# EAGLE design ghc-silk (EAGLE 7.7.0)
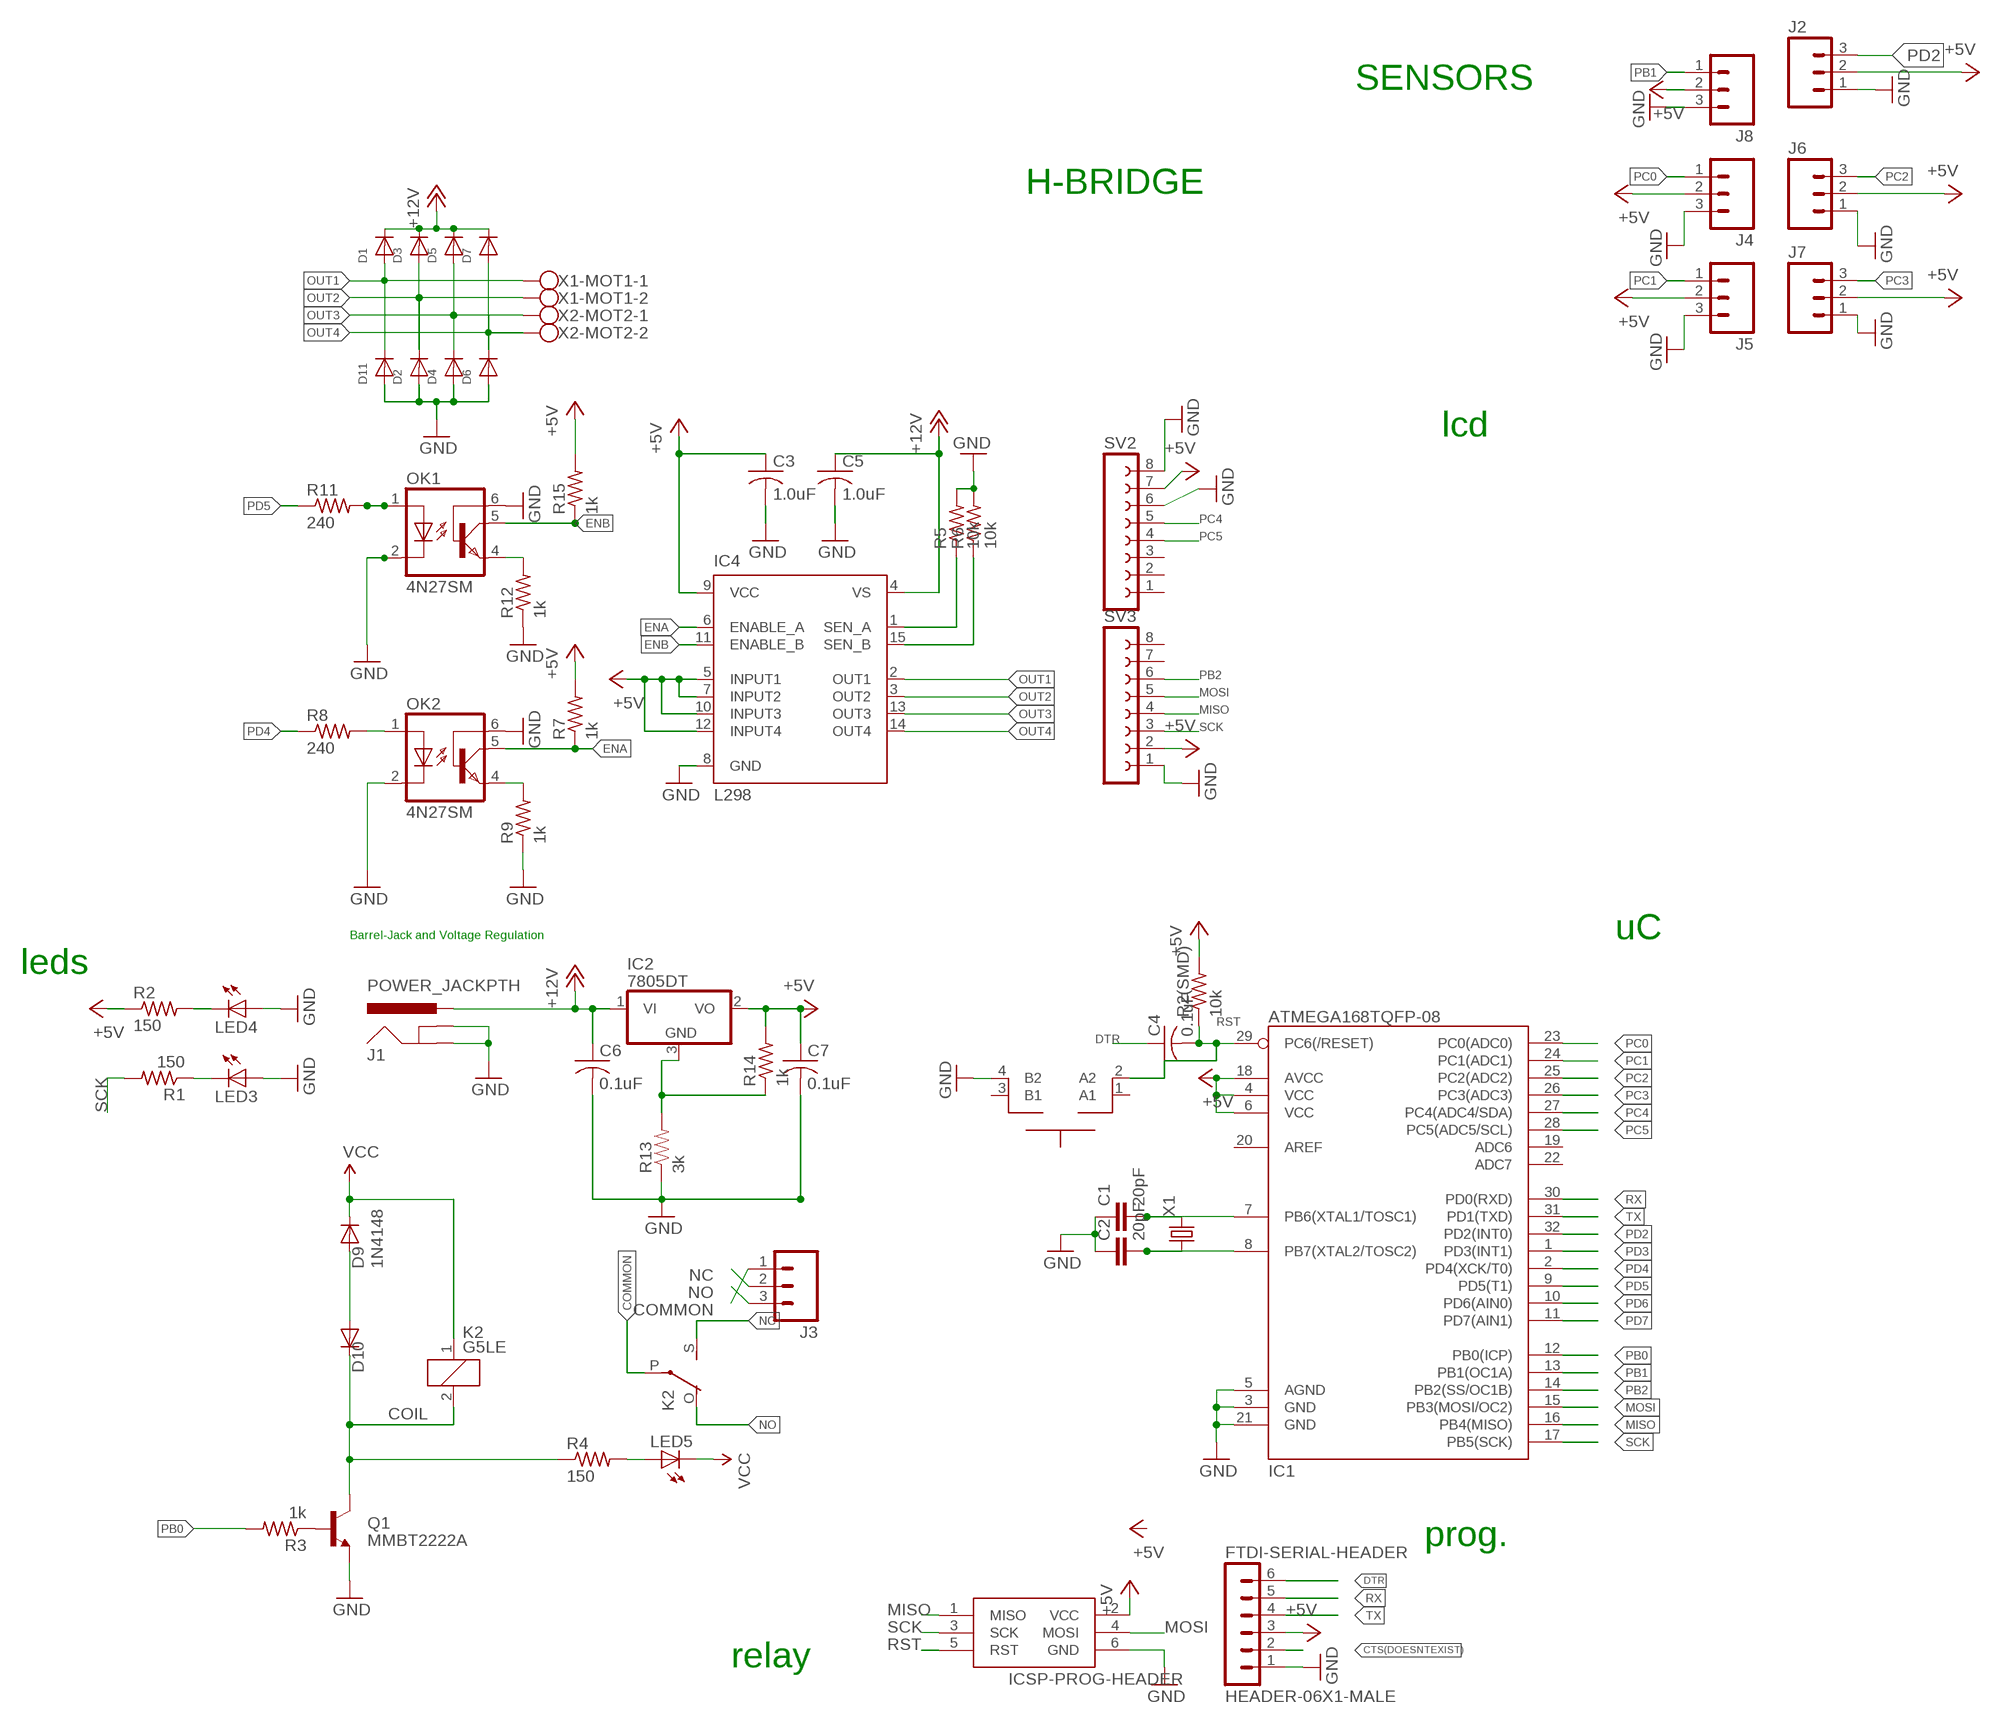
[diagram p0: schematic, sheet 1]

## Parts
C1  20pF  C-EUC0805  [C0805]
C2  20pF  C-EUC0805  [C0805]
C3  1.0uF  C-USC0805  [C0805]
C4  0.1uF  C-USC0805  [C0805]
C5  1.0uF  C-USC0805  [C0805]
C6  0.1uF  C-USC0805  [C0805]
C7  0.1uF  C-USC0805  [C0805]
D1  DIODESOD-523  [SOD-523]
D2  DIODESOD-523  [SOD-523]
D3  DIODESOD-523  [SOD-523]
D4  DIODESOD-523  [SOD-523]
D5  DIODESOD-523  [SOD-523]
D6  DIODESOD-523  [SOD-523]
D7  DIODESOD-523  [SOD-523]
D9  1N4148  DIODESOD-323F  [SOD-323F]
D10  Zener  DIODESOD-323F  [SOD-323F]
D11  DIODESOD-523  [SOD-523]
FTDI-SERIAL-HEADER  HEADER-06X1-MALE  [06X1-PTH]
IC1  ATMEGA168TQFP-08  [TQFP32-08]
IC2  7805DT  [TO252]
IC4  L298  [MULTIWATT-15]
ICSP-PROG-HEADER  AVRISP-6  [AVRISP]
J1  POWER_JACKPTH  [POWER_JACK_PTH]
J2  M03SCREW_LOCK  [SCREWTERMINAL-3.5MM-3_LOCK.007S]
J3  M03-SCREW-5MM  [SCREWTERMINAL-5MM-3]
J4  M03SCREW_LOCK  [SCREWTERMINAL-3.5MM-3_LOCK.007S]
J5  M03SCREW_LOCK  [SCREWTERMINAL-3.5MM-3_LOCK.007S]
J6  M03SCREW_LOCK  [SCREWTERMINAL-3.5MM-3_LOCK.007S]
J7  M03SCREW_LOCK  [SCREWTERMINAL-3.5MM-3_LOCK.007S]
J8  M03SCREW_LOCK  [SCREWTERMINAL-3.5MM-3_LOCK.007S]
K2  G5LE  [G5LE]
LED3  LEDCHIP-LED0805  [CHIP-LED0805]
LED4  LEDCHIP-LED0805  [CHIP-LED0805]
LED5  LEDCHIP-LED0805  [CHIP-LED0805]
OK1  4N27SM  [DIL6-SMD]
OK2  4N27SM  [DIL6-SMD]
Q1  MMBT2222A  TRANSISTOR_NPNMMBT2222A  [SOT23-3]
R1  150  R-US_M0805  [M0805]
R2  150  R-US_M0805  [M0805]
R2(SMD)  10k  R-US_M0805  [M0805]
R3  1k  R-US_M0805  [M0805]
R4  150  R-US_M0805  [M0805]
R5  10k  R-US_M0805  [M0805]
R6  10k  R-US_M0805  [M0805]
R7  1k  R-US_M0805  [M0805]
R8  240  R-US_M0805  [M0805]
R9  1k  R-US_M0805  [M0805]
R11  240  R-US_M0805  [M0805]
R12  1k  R-US_M0805  [M0805]
R13  3k  RESISTOR0402  [0402-RES]
R14  1k  R-US_M0805  [M0805]
R15  1k  R-US_M0805  [M0805]
SV2  FE08-1  [FE08]
SV3  FE08-1  [FE08]
SW2  MOMENTARYBUTTON  [SPST_NO_SMD]
X1  CRYSTALHC49UP  [HC49UP]
X1-MOT1  W237-102  [W237-102]
X2-MOT2  W237-102  [W237-102]

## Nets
+5V: C3.1 C7.1 FTDI-SERIAL-HEADER.3 IC1.4(VCC) IC1.6(VCC) IC1.18(AVCC) IC2.2(VO) IC4.5(INPUT1) IC4.7(INPUT2) IC4.9(VCC) IC4.10(INPUT3) IC4.12(INPUT4) ICSP-PROG-HEADER.2(VCC) J2.2 J4.2 J5.2 J6.2 J7.2 J8.2 R2(SMD).2 R2.1 R7.2 R14.2 R15.2 SV2.7 SV3.2
+12V: C5.1 C6.1 D1.K(C) D3.K(C) D5.K(C) D7.K(C) IC2.1(VI) IC4.4(VS) J1.PWR
COIL: D10.C K2.2 Q1.3(C) R4.1
COMMON: J3.1 K2.P(2:P)
CTS(DOESNTEXIST): FTDI-SERIAL-HEADER.2
DIODENODE: D9.A D10.A
DTR: C4.1 FTDI-SERIAL-HEADER.6
ENA: IC4.6(ENABLE_A) OK2.5(COL) R7.1
ENB: IC4.11(ENABLE_B) OK1.5(COL) R15.1
GND: C1.1 C2.1 C3.2 C5.2 C6.2 C7.2 D2.A D4.A D6.A D11.A FTDI-SERIAL-HEADER.1 IC1.3(GND) IC1.5(AGND) IC1.21(GND) IC4.8(GND) ICSP-PROG-HEADER.6(GND) J1.GND J1.GNDBREAK J2.1 J4.3 J5.3 J6.1 J7.1 J8.3 LED3.A LED4.A OK1.2(C) OK1.6(BAS) OK2.2(C) OK2.6(BAS) Q1.2(E) R5.2 R6.2 R9.1 R12.1 R13.1 SV2.6 SV2.8 SV3.1 SW2.4(B2)
MISO: IC1.16(PB4(MISO)) ICSP-PROG-HEADER.1(MISO) SV3.4
MOSI: IC1.15(PB3(MOSI/OC2)) ICSP-PROG-HEADER.4(MOSI) SV3.5
N$1: OK2.1(A) R8.2
N$2: LED4.C R2.2
N$3: LED5.A R4.2
N$5: OK2.4(EMI) R9.2
N$6: Q1.1(B) R3.1
N$7: IC2.3(GND) R13.2 R14.1
N$8: OK1.1(A) R11.2
N$10: LED3.C R1.1
N$11: C1.2 IC1.7(PB6(XTAL1/TOSC1)) X1.2
N$13: C2.2 IC1.8(PB7(XTAL2/TOSC2)) X1.1
N$15: OK1.4(EMI) R12.2
NC: J3.2 K2.S(2:S)
NO: J3.3 K2.O(2:O)
OUT1: D1.A D11.K(C) IC4.2(OUT1) X1-MOT1.1
OUT2: D2.K(C) D3.A IC4.3(OUT2) X1-MOT1.2
OUT3: D4.K(C) D5.A IC4.13(OUT3) X2-MOT2.1
OUT4: D6.K(C) D7.A IC4.14(OUT4) X2-MOT2.2
PB0: IC1.12(PB0(ICP)) R3.2
PB1: IC1.13(PB1(OC1A)) J8.1
PB2: IC1.14(PB2(SS/OC1B)) SV3.6
PC0: IC1.23(PC0(ADC0)) J4.1
PC1: IC1.24(PC1(ADC1)) J5.1
PC2: IC1.25(PC2(ADC2)) J6.3
PC3: IC1.26(PC3(ADC3)) J7.3
PC4: IC1.27(PC4(ADC4/SDA)) SV2.5
PC5: IC1.28(PC5(ADC5/SCL)) SV2.4
PD2: IC1.32(PD2(INT0)) J2.3
PD3: IC1.1(PD3(INT1))
PD4: IC1.2(PD4(XCK/T0)) R8.1
PD5: IC1.9(PD5(T1)) R11.1
PD6: IC1.10(PD6(AIN0))
PD7: IC1.11(PD7(AIN1))
RST: C4.2 IC1.29(PC6(/RESET)) ICSP-PROG-HEADER.5(RST) R2(SMD).1 SW2.2(A2)
RX: FTDI-SERIAL-HEADER.5 IC1.30(PD0(RXD))
SCK: IC1.17(PB5(SCK)) ICSP-PROG-HEADER.3(SCK) R1.2 SV3.3
SEN_A: IC4.1(SEN_A) R5.1
SEN_B: IC4.15(SEN_B) R6.1
TX: FTDI-SERIAL-HEADER.4 IC1.31(PD1(TXD))
VCC: D9.C K2.1 LED5.C
Unconnected: IC1.19(ADC6) IC1.20(AREF) IC1.22(ADC7) SV2.1 SV2.2 SV2.3 SV3.7 SV3.8 SW2.1(A1) SW2.3(B1)

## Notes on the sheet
- SENSORS
- H-BRIDGE
- lcd
- Barrel-Jack and Voltage Regulation | uC
- leds
- prog.
- relay

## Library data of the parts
C1 C2 = resistor:C-EU: CAPACITOR, European symbol
C3-C7 = adafruit:C-US: CAPACITOR, American symbol
D1-D7 D10 D11 = adafruit:DIODE: Diode
D9 = adafruit:DIODE: Diode; PROD_ID: DIO-08378
FTDI-SERIAL-HEADER = GeekAmmo:HEADER-06X1?: 6 x 0.1 inch Header 40x1 0.1inch Male Breakaway header can be used. - 4UCON 00834 For female part, if possible use 6 x 1 without breaking.; OTHER: 4UCON 00834; URL: http://www.4uconnector.com/online/SearchPro.asp?FormName=ProSearch&FormAction=search&s_GroupNo=&s_keyword=00834
IC1 = atmega328p:ATMEGA168
IC2 = ece388:78*: Positive VOLTAGE REGULATOR Added bigger pads to the TO-92 package
IC4 = st-microelectronics:L298: DUAL FULL-BRIDGE DRIVER; MPN: L298N; OC_FARNELL: 1589425; OC_NEWARK: 32M1527
ICSP-PROG-HEADER = adafruit:AVRISP: AVR ISP HEADER Standard 6 pin header for AVR programming
J1 = SparkFun-Connectors:POWER_JACK: Power Jack This is the standard 5.5mm barrel jack for power. The PTH is the most common, proven, reliable, footprint. The Slot footprint only works if the mill layer is transmitted to the PCB fab house so be warned. Mating wall wart : TOL-00298 (and others); PROD_ID: CONN-08197
J2 J4-J8 = SparkFun-Connectors:M03: Header 3 Standard 3-pin 0.1" header. Use with straight break away headers (SKU : PRT-00116), right angle break away headers (PRT-00553), swiss pins (PRT-00743), machine pins (PRT-00117), and female headers (PRT-00115). Molex polarized connector foot print use with SKU : PRT-08232 with associated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; PROD_ID: CONN-08288
J3 = SparkFun-Connectors:M03: Header 3 Standard 3-pin 0.1" header. Use with straight break away headers (SKU : PRT-00116), right angle break away headers (PRT-00553), swiss pins (PRT-00743), machine pins (PRT-00117), and female headers (PRT-00115). Molex polarized connector foot print use with SKU : PRT-08232 with associated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; PROD_ID: CONN-10134; STOREFRONT_ID: PRT-08433
K2 = relay:G5LE: RELAY 1 x switch, 10 A/120 V AC, 8 A/30 V DC, Omron; OC_FARNELL: unknown; OC_NEWARK: unknown
LED3-LED5 = adafruit:LED: LED
OK1 OK2 = optocoupler:4N*?M: General Purpose 6-Pin Phototransistor Optocouplers Source: http://www.fairchildsemi.com/ds/4N/4N35-M.pdf; MF: FAIRCHILD SEMICONDUCTOR; MPN: 4N27S-M; OC_FARNELL: unknown; OC_NEWARK: 05C3300
Q1 = SparkFun-DiscreteSemi:TRANSISTOR_NPN: Generic NPN BJT MMBT2222A - TRANS-08049 (SOT-23, 1A 40V) MPSA42 - TRANS-09116 (SOT-23, 500mA 300V) MMBT5088LT1G - TRANS-11160 (SOT-23, 50 mA 30V) BC547 - COM-08928 (TO-92 45V 100mA) (1.Collector 2.Base 3.Emitter) 2N3904 - COM-00521 (TO-92 40V 200mA) (1.Emitter 2.Base 3.Collector) P2N2222A -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; PROD_ID: TRANS-08049
R1 R2 R2(SMD) R3-R9 R11 R12 R14 R15 = adafruit:R-US_: RESISTOR, American symbol
R13 = SparkFun-Resistors:RESISTOR: Resistor
SV2 SV3 = con-lsta:FE08-1: FEMALE HEADER; OC_FARNELL: unknown; OC_NEWARK: unknown
SW2 = ece388:MOMENTARYBUTTON
X1 = adafruit:CRYSTAL: CRYSTAL; OC_FARNELL: unknown; OC_NEWARK: unknown
X1-MOT1 X2-MOT2 = con-wago-500:W237-102: WAGO SCREW CLAMP; MPN: 237-102; OC_FARNELL: unknown; OC_NEWARK: 70K9898

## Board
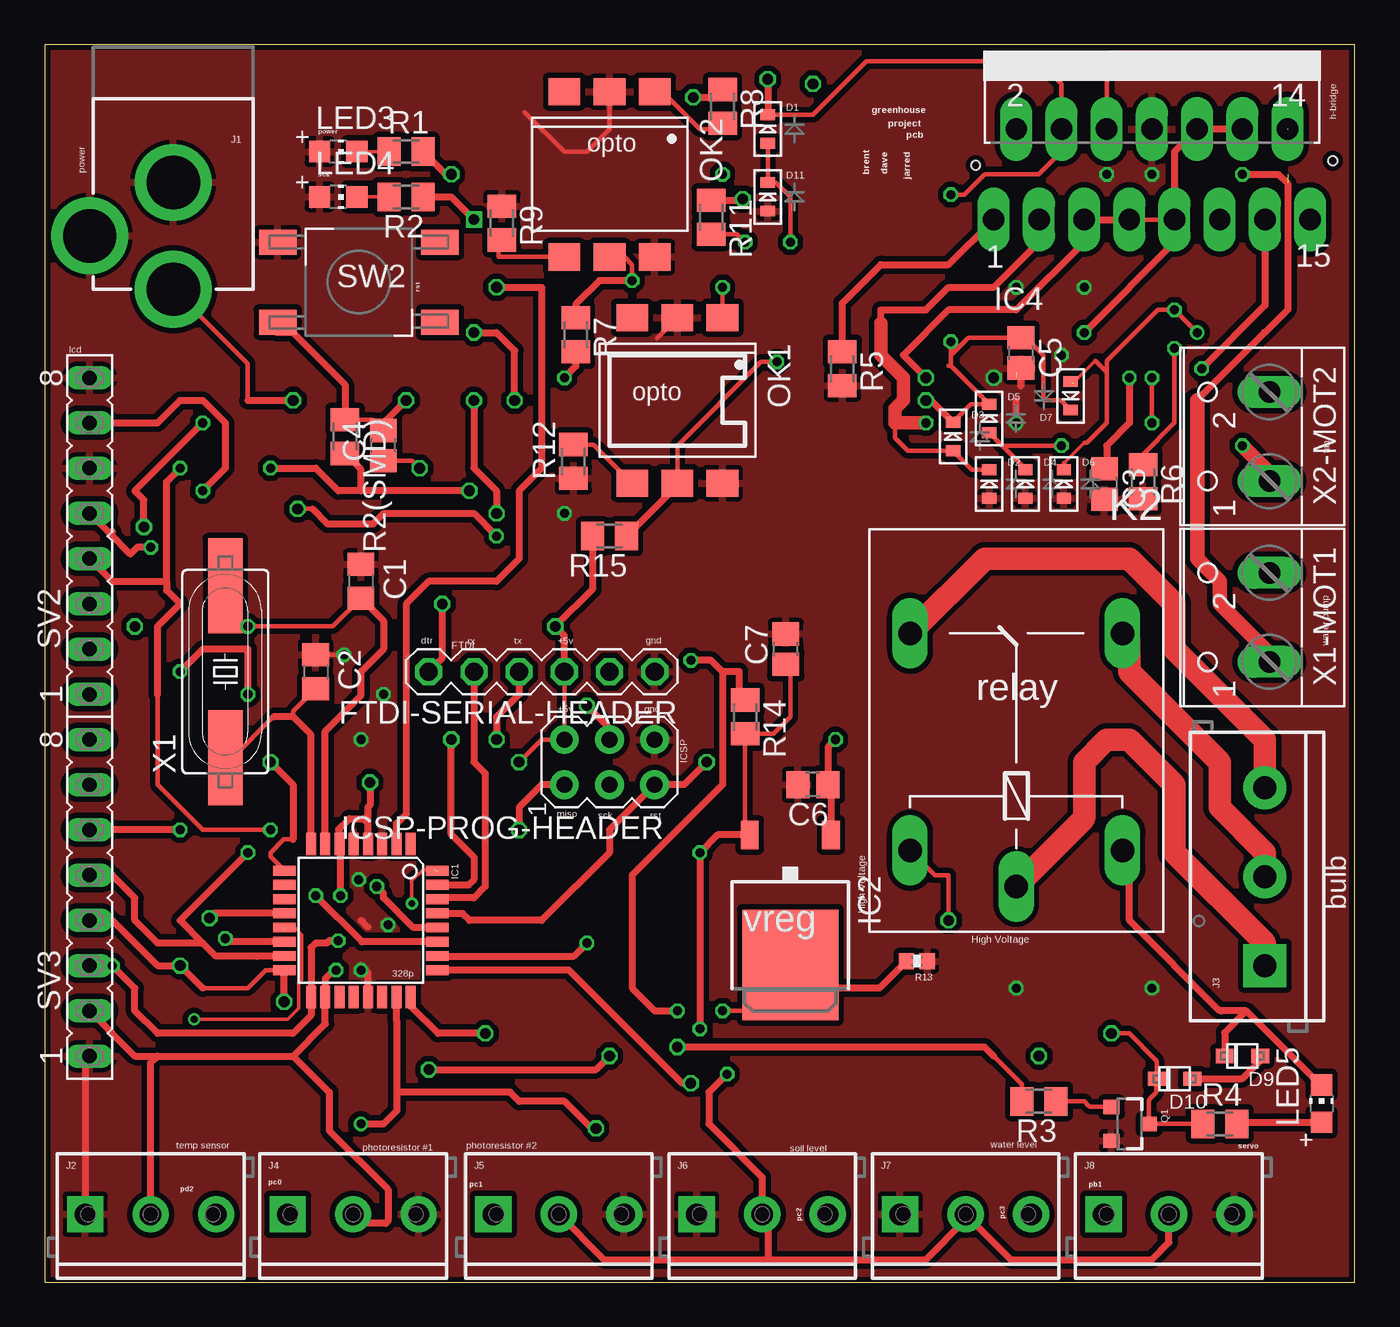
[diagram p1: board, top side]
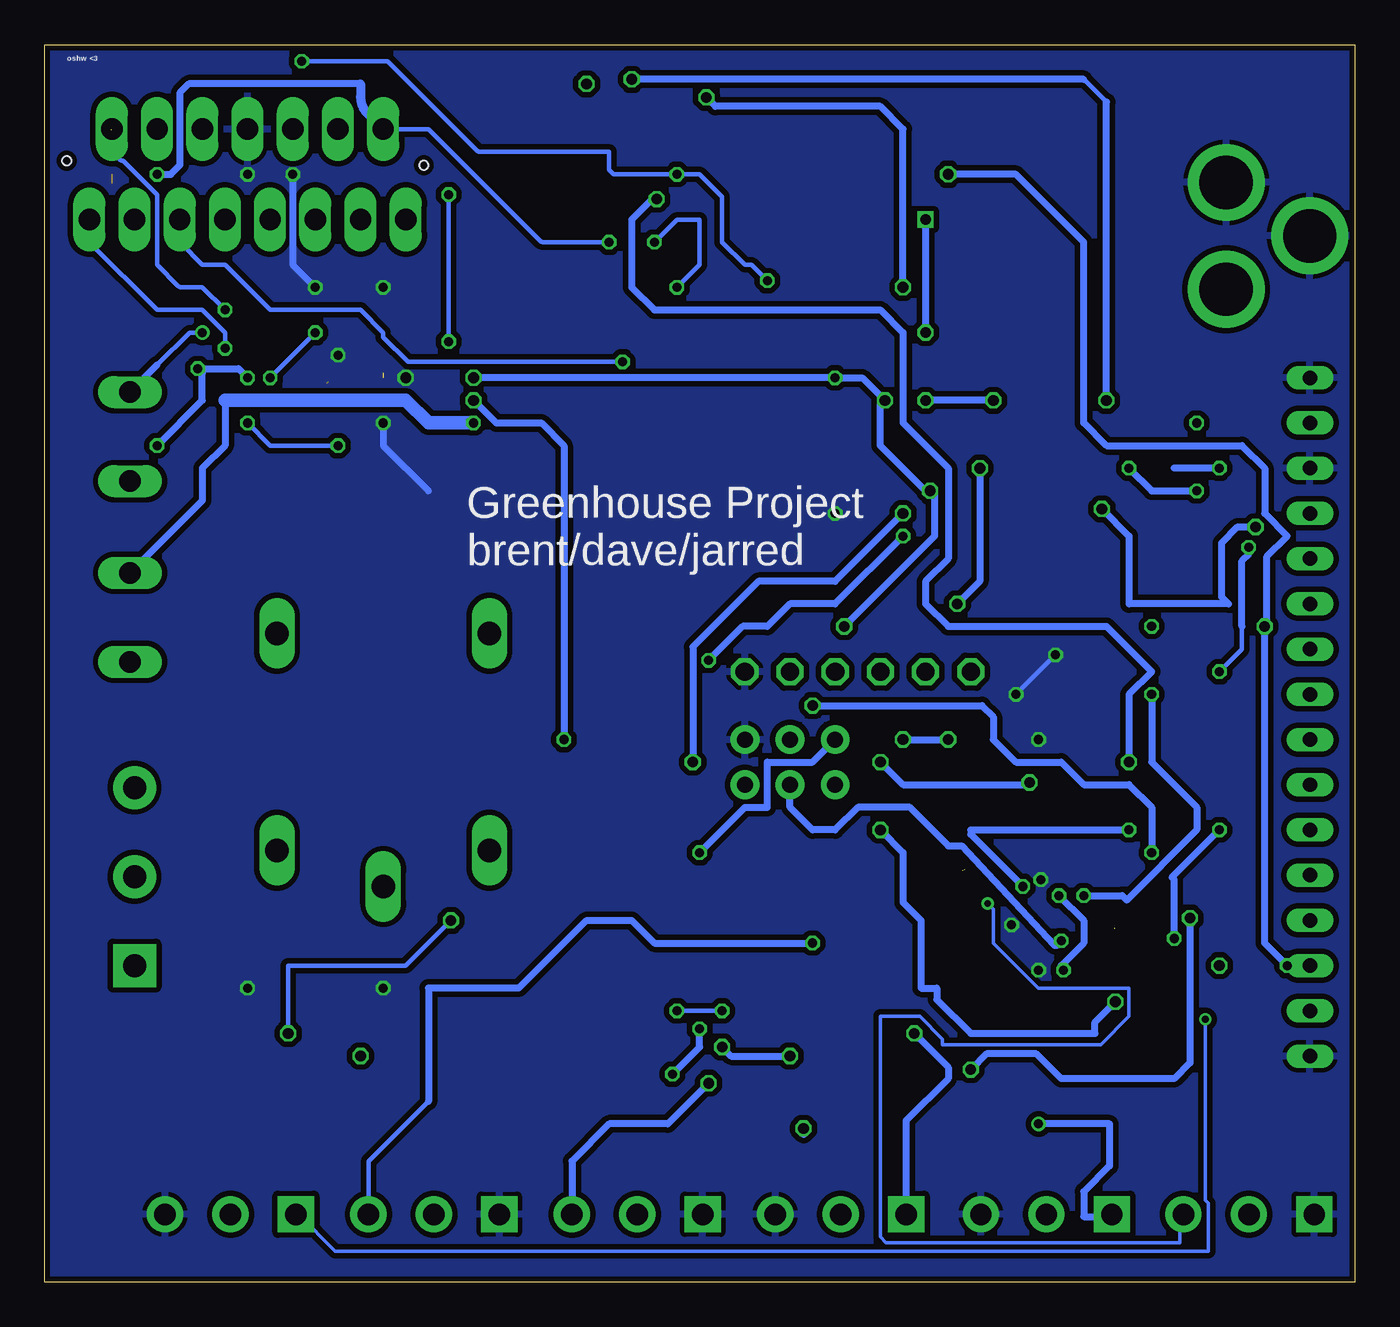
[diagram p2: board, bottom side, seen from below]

Size 73.64 x 69.52 mm. Coordinates in mm from the lower left corner, seen from the top.
Outline: 0,0 73.64,0 73.64,69.52 0,69.52 0,0
Copper layers (1*16): Top 0.035mm / dielectric 1.5mm / Bottom 0.035mm
Design rules "Dirty8TS *": minimum track width 8mil, minimum drill 15mil, track to track 8mil, track to pad 8mil, pad to pad 8mil, via to via 8mil, smd to smd 0mil, copper to edge 10mil, drill to drill 10mil, minimum pad ring 10mil, minimum via ring 6mil, stop-mask expansion 2mil, vias tented up to drill 25mil, thermal gap 10mil
Holes 0.51 mm at 52.32,62.74 72.39,62.99

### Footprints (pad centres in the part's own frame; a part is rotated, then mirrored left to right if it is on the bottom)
C0805 = smd 1.3 x 1.5: 1 -0.95,0; 2 0.95,0
C0805' = smd 1.3 x 1.5: 1 -0.85,0; 2 0.85,0
SOD-523 = smd 0.8 x 0.6: A 0,-0.8; K 0,0.8
SOD-323F = smd 1 x 0.8: A -1,0; C 1,0
06X1-PTH = drill 1.016 octagon: 1 -6.35,0; 2 -3.81,0; 3 -1.27,0; 4 1.27,0; 5 3.81,0; 6 6.35,0
TQFP32-08 = smd 1.27 x 0.559: 1 -4.293,2.8; 2 -4.293,2; 3 -4.293,1.2; 4 -4.293,0.4; 5 -4.293,-0.4; 6 -4.293,-1.2; 7 -4.293,-2; 8 -4.293,-2.8; 17 4.293,-2.8; 18 4.293,-2; 19 4.293,-1.2; 20 4.293,-0.4; 21 4.293,0.4; 22 4.293,1.2; 23 4.293,2; 24 4.293,2.8 | smd 0.559 x 1.27: 9 -2.8,-4.293; 10 -2,-4.293; 11 -1.2,-4.293; 12 -0.4,-4.293; 13 0.4,-4.293; 14 1.2,-4.293; 15 2,-4.293; 16 2.8,-4.293; 25 2.8,4.293; 26 2,4.293; 27 1.2,4.293; 28 0.4,4.293; 29 -0.4,4.293; 30 -1.2,4.293; 31 -2,4.293; 32 -2.8,4.293
TO252 = smd 1 x 1.6: 1 -2.28,-4.8; 2 2.28,-4.8 | smd 5.4 x 6.2: 3 0,2.5
MULTIWATT-15 = drill 1.2 long: 1 -8.89,-7.62; 2 -7.62,-2.54; 3 -6.35,-7.62; 4 -5.08,-2.54; 5 -3.81,-7.62; 6 -2.54,-2.54; 7 -1.27,-7.62; 8 0,-2.54; 9 1.27,-7.62; 10 2.54,-2.54; 11 3.81,-7.62; 12 5.08,-2.54; 13 6.35,-7.62; 14 7.62,-2.54; 15 8.89,-7.62
AVRISP = drill 0.9 pad 1.626: 1 -1.27,2.54; 2 1.27,2.54; 3 -1.27,0; 4 1.27,0; 5 -1.27,-2.54; 6 1.27,-2.54
POWER_JACK_PTH = drill 2.997 pad 4.318: GND 0,7.7; GNDBREAK 4.7,10.7; PWR 0,13.7
SCREWTERMINAL-3.5MM-3_LOCK.007S = drill 1.2 pad 2.032 square: 1 -0.178,0 | drill 1.2 pad 2.032: 2 3.5,0; 3 7.178,0
SCREWTERMINAL-5MM-3 = drill 1.3 pad 2.413 square: 1 0,0 | drill 1.3 pad 2.413: 2 5,0; 3 10,0
G5LE = drill 1.321 long: 1 -7.493,-5.969; 2 -7.493,5.969; O 4.699,5.969; P -9.525,0; S 4.699,-5.969
CHIP-LED0805 = smd 1.2 x 1.2: A 0,-1.05; C 0,1.05
DIL6-SMD = smd 1.78 x 1.52: 1 -2.54,-4.645; 2 0,-4.645; 3 2.54,-4.645; 4 2.54,4.645; 5 0,4.645; 6 -2.54,4.645
SOT23-3 = smd 0.8 x 0.9: 1 -0.95,-1; 2 0.95,-1; 3 0,1.1
M0805 = smd 1.3 x 1.6: 1 -0.95,0; 2 0.95,0
0402-RES = smd 0.85 x 0.9: 1 -0.58,0; 2 0.58,0
FE08 = drill 0.813 long: 1 -8.89,0; 2 -6.35,0; 3 -3.81,0; 4 -1.27,0; 5 1.27,0; 6 3.81,0; 7 6.35,0; 8 8.89,0
SPST_NO_SMD = smd 2.108 x 1.397: 1 0,4.496; 2 9.119,4.496; 3 0,0; 4 9.119,0
HC49UP = smd 5.334 x 1.93: 1 -4.826,0; 2 4.826,0
W237-102 = drill 1.194 long: 1 -2.5,-1.27; 2 2.5,-1.27

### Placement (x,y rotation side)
C1  17.78,39.37 270 top
C2  15.24,34.29 270 top
C3  1.0uF  [C0805']  59.56,44.83 270 top
C4  0.1uF  [C0805']  19.05,46.99 90 top
C5  1.0uF  [C0805']  54.86,52.2 270 top
C6  0.1uF  [C0805']  43.18,27.94 180 top
C7  0.1uF  [C0805']  41.66,35.56 90 top
D1  40.64,64.77 0 top
D2  53.09,44.83 0 top
D3  51.05,47.5 0 top
D4  55.12,44.83 0 top
D5  53.09,48.51 0 top
D6  57.28,44.83 0 top
D7  57.66,49.78 180 top
D9  67.31,12.7 180 top
D10  63.5,11.43 180 top
D11  40.64,60.96 0 top
FTDI-SERIAL-HEADER  27.94,34.29 180 top
IC1  17.78,20.32 270 top
IC2  41.91,20.32 180 top
IC4  62.23,67.31 0 top
ICSP-PROG-HEADER  31.75,29.21 90 top
J1  7.24,69.47 180 top
J2  2.46,3.81 0 top
J3  68.58,17.78 90 top
J4  13.84,3.81 0 top
J5  25.4,3.81 0 top
J6  36.83,3.81 0 top
J7  48.26,3.81 0 top
J8  59.69,3.81 0 top
K2  54.61,31.75 90 top
LED3  16.51,63.5 270 top
LED4  16.51,60.96 270 top
LED5  71.75,10.03 0 top
OK1  35.56,49.53 180 top
OK2  31.75,62.23 180 top
Q1  60.96,8.89 270 top
R1  20.32,63.5 0 top
R2  20.32,60.96 180 top
R2(SMD)  16.89,47.5 270 top
R3  55.88,10.16 180 top
R4  66.04,8.89 0 top
R5  44.83,51.31 270 top
R6  61.72,44.96 270 top
R7  29.84,53.21 270 top
R8  38.1,66.04 270 top
R9  25.7,59.49 270 top
R11  37.47,59.82 270 top
R12  29.72,46.1 90 top
R13  49.02,18.03 180 top
R14  39.37,31.75 270 top
R15  31.75,41.91 180 top
SV2  2.54,41.91 90 top
SV3  2.54,21.59 90 top
SW2  22.23,58.42 180 top
X1  10.16,34.29 90 top
X1-MOT1  67.56,37.34 90 top
X2-MOT2  67.56,47.5 90 top

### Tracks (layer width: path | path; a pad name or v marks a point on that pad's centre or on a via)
+5V  (via drill 0.51, 0.6)
  Top 0.254: v26.67,29.21 27.94,30.48 ICSP-PROG-HEADER.2 FTDI-SERIAL-HEADER.3 | IC4.9 IC4.7 | IC2.2 39.37,25.38 R14.2 40.96,30.8 41.91,31.75 41.91,34.46 C7.1
  Top 0.406: v23.88,44.45 17.78,44.45 | IC1.6 16.58,25.33 16.51,25.4 17.14,26.04 17.91,26.04 18.16,25.78 | 18.16,25.78 18.16,24.63 IC1.4 18.18,25.8 | v49.53,50.8 48.26,52.07 50.8,54.61 54.61,54.61 58.42,58.42 IC4.5 IC4.7 | IC2.2 37.82,25.12 v36.83,24.13 v36.83,14.22 | IC4.12 IC4.10 63.5,63.5 IC4.9 63.5,58.42 v58.42,53.34 | 18.16,25.78 18.16,26.67 18.29,26.8 v18.29,28.07 | FTDI-SERIAL-HEADER.3 29.21,36.32 v28.7,36.83 30.8,38.93 R15.2 | v38.35,11.68 37.34,10.67 37.34,8.89 40.33,5.9 J6.2 40.64,3.5 40.64,1.27 | 17.78,44.45 17.78,45.66 R2(SMD).2 | v12.7,45.72 15.24,45.72 16.51,44.45 17.78,44.45 | R2.1 22.86,60.96 v24.13,59.69 | v24.13,53.34 25.4,53.34 26.42,52.32 v26.42,49.53 | v60.96,50.8 60.96,48.26 59.69,46.99 59.69,45.81 C3.1 | R7.2 29.84,51.44 v29.21,50.8 | SV2.7 6.35,48.26 7.62,49.53 8.89,49.53 10.16,48.26 10.16,45.72 v8.89,44.45 | 13.97,12.7 15.78,14.51 IC1.18 15.78,17.05 16.26,17.53 v16.38,17.53 | SV3.2 5.08,12.7 6.35,12.7 | 6.35,12.7 13.97,12.7 | IC1.6 16.51,24.54 | v16.64,21.72 16.64,24.56 IC1.6 | J2.2 5.96,12.31 6.35,12.7 | J4.2 17.85,3.3 19.18,3.3 19.3,3.43 19.3,5.21 16,8.51 16,10.67 13.97,12.7 | 40.64,1.27 49.53,1.27 51.76,3.5 J7.2 54.3,1.27 62.23,1.27 63.19,2.23 J8.2 | J5.2 31.44,1.27 40.64,1.27
  Bottom 0.254: v60.96,50.8 v58.42,53.34
  Bottom 0.406: v28.7,36.83 23.62,41.91 23.62,44.2 v23.88,44.45 24.13,44.45 26.67,46.99 26.67,49.28 v26.42,49.53 27.69,50.8 v29.21,50.8 v49.53,50.8 | v38.35,11.68 36.83,13.21 v36.83,14.22 | v12.7,45.72 11.43,44.45 v8.89,44.45 | v24.13,59.69 v24.13,53.34 | v36.83,24.13 34.29,26.67 33.02,26.67 33.02,29.21 30.48,29.21 ICSP-PROG-HEADER.2 | v16.64,21.72 15.24,20.32 15.24,19.05 16.51,17.78 16.38,17.65 v16.38,17.53 | v26.67,29.21 25.4,27.94 18.41,27.94 v18.29,28.07
+12V  (via drill 0.51, 0.6)
  Top 0.254: D1.K 43.18,65.57 46.19,68.58 55.88,68.58 57.15,67.31 IC4.4 57.15,63.5 55.88,62.23 52.94,62.23 arc45 52.76,62.16 51.69,61.09 v50.93,61.09 | v50.93,52.83 50.93,52.07 | 50.93,52.07 50.93,51.6 50.8,51.47 50.93,51.47 D5.K 52.07,49.31 D3.K | D7.K 57.11,49.53 56.13,49.53 56.13,52.07 55.16,53.05 C5.1 51.9,53.05 50.93,52.07 | 11.43,49.53 11.43,51.58 J1.PWR
  Top 0.406: 11.43,49.53 v13.97,49.53 | v40.64,67.56 D1.K | D3.K 49.82,49.53 v49.53,49.53 | IC2.1 44.19,27.78 C6.1 44.03,30.06 v44.45,30.48
  Bottom 0.254: 15.24,67.56 13.97,66.29 | v50.93,52.83 v50.93,61.09
  Bottom 0.406: v13.97,49.53 13.97,66.29 | 15.24,67.56 v40.64,67.56 | v49.53,49.53 48.26,48.26 45.72,48.26 44.45,46.99 v44.45,30.48
COIL  (via drill 0.6)
  Top 0.254: v50.8,20.32 50.8,22.86 50.04,22.86 K2.2 | R4.1 Q1.3 62.06,10.14 arc-45 62.13,10.32 62.48,10.67 62.48,11.39 arc-45 D10.C 62.5,12.32 arc45 62.43,12.5 60.96,13.97 v59.94,13.97
  Bottom 0.254: v50.8,20.32 53.34,17.78 59.94,17.78 v59.94,13.97
COMMON
  Top 1.27: K2.P 58.35,25.96 arc45 58.42,26.14 58.42,29.21 59.62,30.41 arc-45 59.8,30.48 60.96,30.48 63.5,27.94 63.5,24.13 68.51,19.12 arc-45 68.58,18.95 J3.1
DIODENODE
  Top 0.406: D10.A 67.31,11.43 68.31,12.43 D9.A
DTR  (via drill 0.6)
  Top 0.254: C4.1 20.66,46.14 v21.08,45.72
  Top 0.406: v22.35,38.1 22.35,35.05 FTDI-SERIAL-HEADER.6
  Bottom 0.406: v21.08,45.72 21.08,39.37 v22.35,38.1
ENA  (via drill 0.51)
  Top 0.254: OK2.5 32.59,57.59 33.02,57.15 v33.02,56.26 | IC4.6 59.69,67.97 arc45 59.62,68.15 v59.18,68.58
  Top 0.406: v33.02,56.26 31.18,56.26 29.84,54.92 R7.1
  Bottom 0.254: v59.18,68.58 54.36,68.58 49.35,63.57 arc-45 49.17,63.5 41.91,63.5 41.91,62.48 41.66,62.23 v38.1,62.23 36.83,62.23 35.56,60.96 35.56,58.42 34.29,57.15 33.91,57.15 v33.02,56.26
ENB  (via drill 0.51)
  Top 0.254: OK1.5 35.56,46.99 40.26,51.69 v41.15,51.69
  Top 0.406: OK1.5 35.56,44.77 R15.1
  Bottom 0.254: v41.15,51.69 53.21,51.69 54.61,53.09 54.61,53.34 55.88,54.61 60.96,54.61 63.5,57.15 64.77,57.15 65.97,58.35 arc45 66.04,58.52 IC4.11
GND  (via drill 0.51, 0.6)  (1 unrouted)
  Top 0.203: LED4.A 15.09,60.59 arc45 15.01,60.41
  Top 0.254: 59.51,44.03 C3.2 | 61.7,43.98 R6.2 | OK2.2 31.75,64.77 30.48,63.5 29.21,63.5 26.99,65.72 | 34.41,53.02 OK1.2 | C2.1 v16.83,35.24
  Top 0.406: 54.86,50.33 C5.2 54.61,51.09 | LED3.A 15.24,63.72 | J5.3 33.02,3.81 | v54.61,48.26 54.61,49.53 | v17.65,22.61 17.78,22.48 | v17.78,17.53 18.18,17.13 | IC1.21 18.18,17.13 | 18.18,17.13 18.18,17.38 17.78,17.78 | 18.16,19.94 17.78,20.32 | SV3.1 2.29,12.7 J2.1
  Bottom 0.254: v16.83,35.24 v19.05,33.02
  Bottom 0.406: v54.61,48.26 54.61,46.99 52.07,44.45 | v59.69,62.23 59.69,57.15 v58.42,55.88
  other vias: 53.34,50.8 62.23,16.51 29.21,43.18 19.3,20.07 54.61,16.51 17.78,30.48 62.23,62.23 57.15,52.07 54.61,55.88
  pour Top (isolate 0.305): 0,69.85 73.66,69.85 73.66,0 0,0
  pour Bottom (isolate 0.305): 0,69.85 73.66,69.85 73.66,0 0,0
MISO  (via drill 0.6)
  Top 0.254: 8.89,16.51 11.43,16.51 12.44,17.52 IC1.16
  Top 0.406: ICSP-PROG-HEADER.1 27.94,27.94 26.67,26.67 v26.67,25.4 | v13.46,15.75 13.46,17.5 IC1.16 | 8.89,16.51 v7.62,17.78 6.35,17.78 3.81,20.32 SV3.4
  Bottom 0.406: v26.67,25.4 25.4,24.13 25.4,21.34 24.38,20.32 24.38,16.51 23.5,16.51 23.5,15.88 21.59,13.97 14.61,13.97 14.61,14.61 v13.46,15.75
MOSI  (via drill 0.51, 0.6)
  Top 0.406: ICSP-PROG-HEADER.4 31.75,31.11 v30.48,32.38 | IC1.15 11.97,18.32 | 11.97,18.32 11.94,18.29 | SV3.5 3.81,22.86 5.08,21.59 5.08,20.32 6.35,19.05 8.89,19.05 | v11.43,24.13 7.62,20.32 8.89,19.05 | 11.97,18.32 9.62,18.32 8.89,19.05
  Bottom 0.406: v30.48,32.38 20.95,32.38 20.32,31.75 20.32,30.48 19.05,29.21 16.51,29.21 15.24,27.94 12.7,27.94 11.43,26.67 v11.43,24.13
N$1
  Top 0.254: R8.2 37.78,64.77 36.83,64.77 34.73,66.88 OK2.1
N$2
  Top 0.203: LED4.C R2.2
N$3
  Top 0.406: R4.2 67.08,8.98 LED5.A
N$5
  Top 0.254: OK2.4 25.52,57.59 25.52,58.35 R9.2
N$6
  Top 0.254: Q1.1 58.84,9.84 arc-45 58.67,9.91 58.42,10.16 R3.1
N$7  (via drill 0.51, 0.6)
  Top 0.254: v38.1,15.24 39.33,15.24 41.26,17.16 IC2.3 | 15.06,43.43 v14.22,43.43
  Top 0.406: v25.4,41.91 24.13,43.18 19.05,43.18 18.47,42.6 15.89,42.6 15.06,43.43 | 38.1,34.29 38.1,27.94 33.02,22.86 33.02,16.51 34.29,15.24 v35.56,15.24 | v8.89,48.26 5.08,44.45 5.59,43.94 v5.59,42.42 | 38.1,34.29 37.47,34.92 v36.32,34.92 | R13.2 46.92,16.51 41.91,16.51 41.26,17.16 | 38.1,34.29 39.05,34.29 39.05,33.02 R14.1
  Bottom 0.254: v35.56,15.24 v38.1,15.24
  Bottom 0.406: v14.22,43.43 12.7,41.91 12.7,38.1 7.11,38.1 7.49,38.48 7.49,41.53 6.6,42.42 v5.59,42.42 | v25.4,41.91 29.21,38.1 31.75,38.1 33.02,36.83 34.42,36.83 v36.32,34.92
N$8  (via drill 0.51)
  Top 0.254: OK1.1 v38.1,55.88 | v39.37,58.42 38.92,58.87 R11.2
  Bottom 0.254: v38.1,55.88 36.83,57.15 36.83,59.69 38.1,59.69 v39.37,58.42
N$10
  Top 0.203: LED3.C R1.1
N$11  (via drill 0.51)
  Top 0.254: C1.2 16.19,36.83 v11.43,36.83 10.16,36.83 X1.2
  Top 0.406: IC1.7 15.78,30.95 17.78,32.95 17.78,34.29 19.05,35.56 19.05,37.15 C1.2
N$13
  Top 0.254: 12.86,31.75 10.57,29.46 | C2.2 13.97,32.07 13.97,31.75
  Top 0.406: IC1.8 14.98,30.74 13.97,31.75 12.86,31.75 | 10.57,29.46 X1.1
N$14  (via drill 0.6)
  other vias: 55.88,12.7
N$15
  Top 0.254: R12.2 30.85,47.05 OK1.4
N$16  (via drill 0.6)
  other vias: 43.18,67.31
NC
  Top 1.27: J3.2 68.58,24.13 66.04,26.67 66.04,29.21 60.96,34.29 60.96,36.07 K2.S
NO
  Top 1.27: K2.O 52.83,40.64 60.96,40.64 63.5,38.1 63.5,35.56 68.58,30.48 J3.3
OUT1  (via drill 0.51)  (1 unrouted)
  Top 0.254: D1.A D11.K 41.11,61.76 41.91,60.96 v41.91,58.42 | 64.77,49.57 64.77,49.53
  Top 0.406: 64.77,49.57 68.54,53.34 arc45 68.61,53.37 69.85,54.61 69.85,61.72 69.34,62.23 v67.31,62.23
  Top 0.813: 64.77,49.53 64.77,40.64 66.04,39.37 66.04,38.1 68.79,35.35 68.79,34.8 X1-MOT1.1
  Bottom 0.254: v41.91,58.42 45.62,58.42 arc45 45.79,58.49 52.07,64.77 IC4.2
  Bottom 0.406: 55.88,67.31 65.53,67.31 66.04,66.8 66.04,62.74 66.55,62.23 v67.31,62.23
  Bottom 0.508: 55.88,67.31 55.88,66.57 arc-45 55.51,65.67 IC4.2
OUT2  (via drill 0.51)
  Top 0.254: D2.K 52.12,45.63 D3.A 48.51,46.7 47.79,47.42 47.79,48.26
  Top 0.406: 46.99,53.87 46.99,54.61 49.53,54.61 50.8,55.88 53.34,55.88 55.88,58.42 IC4.3
  Top 0.762: v49.53,48.26 47.79,48.26 47.79,49.06 48.26,49.53 48.26,50.8 46.99,52.07 46.99,53.87
  Bottom 0.254: X1-MOT1.2 68.79,39.88
  Bottom 0.406: 63.5,49.53 63.5,46.99 64.77,45.72 64.77,43.9 X1-MOT1.2
  Bottom 0.762: 63.5,49.53 53.34,49.53 52.07,48.26 v49.53,48.26
OUT3  (via drill 0.51)
  Top 0.254: D4.K 55.12,45.68 D5.A 53.81,46.99 v57.15,46.99 | v62.23,48.26 v62.23,50.8
  Top 0.406: IC4.13 68.58,54.86 v65.02,51.31
  Top 0.813: X2-MOT2.1 68.83,45.47 v67.31,46.99
  Bottom 0.254: v62.23,48.26 60.96,46.99 v57.15,46.99
  Bottom 0.406: v62.23,50.8 62.74,51.31 v65.02,51.31 64.77,51.05 64.77,49.53 v67.31,46.99
OUT4  (via drill 0.51)  (2 unrouted)
  Top 0.203: 58.42,47.15 57.31,46.04 | 57.78,50.48 59.05,51.75
  Top 0.254: D7.A 57.7,50.55 | 57.31,46.04 57.28,46.01 D6.K | 59.05,51.75 59.69,51.12 | 59.69,51.12 59.69,48.26 58.58,47.15 58.42,47.15 | 59.69,51.12 59.69,51.75 62.55,54.61 v63.5,54.61 v64.77,53.34
  Bottom 0.254: 69.89,64.73 69.89,63.54 69.42,63.07 arc-45 69.24,62.99 69.22,62.99 67.31,61.09 67.31,57.15 66.11,55.95 arc-45 65.94,55.88 64.77,55.88 v63.5,54.61 | v64.77,53.34 65.49,53.34 67.31,51.52
  Bottom 0.406: 67.31,51.52 X2-MOT2.2
PB0  (via drill 0.6)
  Top 0.254: 53.34,12.7 54.93,11.11 R3.2
  Top 0.406: IC1.12 9.54,20.72 v9.27,20.45 | v21.59,11.94 30.99,11.94 v31.75,12.7 | 53.34,12.7 52.83,13.21 v35.56,13.21
  Bottom 0.406: v21.59,11.94 20.7,12.83 17.91,12.83 16.51,11.43 10.16,11.43 9.27,12.32 v9.27,20.45 | v35.56,13.21 35.05,12.7 v31.75,12.7
PB1  (via drill 0.38)  (1 unrouted)
  Top 0.203: 13.49,19.84 14.13,19.84 14.45,19.53 14.45,16.99 14.29,16.83 14.29,15.4 13.65,14.76 v8.41,14.76
  Bottom 0.203: v8.41,14.76 8.41,4.6 8.26,4.45 8.26,1.75 57.31,1.75 59.37,3.81 J8.1
PB2  (via drill 0.51)
  Top 0.406: IC1.14 10.23,19.12 10.23,19.23 v10.16,19.3 | v7.62,25.4 SV3.6
  Bottom 0.406: v7.62,25.4 10.29,22.73 10.16,22.61 v10.16,19.3
PC0  (via drill 0.51, 0.6)
  Top 0.406: 19.81,10.67 26.16,10.67 26.67,10.16 29.21,10.16 30.73,8.64 v30.99,8.64 | IC1.23 19.78,14.7 19.81,14.67 19.81,10.67 | v17.78,8.89 19.05,8.89 19.81,9.65 19.81,10.67
  Bottom 0.406: 30.99,8.28 v30.99,8.64 | v17.78,8.89 13.79,8.89 13.79,6.53 15.24,5.08 15.24,3.68 13.79,3.68 J4.1
PC1  (via drill 0.6)
  Top 0.406: IC1.24 20.58,15.5 22.11,13.97 v24.77,13.97
  Bottom 0.406: v24.77,13.97 22.86,12.06 22.86,11.43 25.22,9.07 J5.1
PC2  (via drill 0.6)
  Top 0.406: v36.32,11.18 35.81,11.18 29.47,17.52 IC1.25
  Bottom 0.406: v36.32,11.18 38.61,8.89 41.91,8.89 44.01,6.79 J6.3
PC3  (via drill 0.51)
  Top 0.406: IC1.26 29.75,18.32 v30.48,19.05
  Bottom 0.254: 52.07,10.16 55.44,6.79 J7.3
  Bottom 0.406: 52.07,10.16 52.07,16.51 46.99,16.51 43.18,20.32 40.64,20.32 39.37,19.05 v30.48,19.05
PC4  (via drill 0.51)
  Top 0.406: v11.43,33.02 11.43,35.56 8.89,35.56 v7.62,34.29 | 3.68,42.04 SV2.5 | v15.24,21.72 17.84,19.12 IC1.27 | 3.81,42.16 3.68,42.04 | 3.68,42.04 4.83,40.89 5.21,41.27 v5.97,41.27
  Bottom 0.254: 6.35,36.83 6.35,35.56 v7.62,34.29
  Bottom 0.406: v11.43,33.02 11.43,29.21 8.89,26.67 8.89,25.4 12.83,21.46 13.08,21.72 v15.24,21.72 | 6.35,36.83 6.35,40.51 5.97,40.89 v5.97,41.27
PC5  (via drill 0.51)
  Top 0.254: 6.35,33.02 6.35,27.94 8.89,25.4 v12.7,25.4
  Top 0.406: IC1.28 20.72,19.92 19.05,21.59 19.05,21.84 v18.67,22.23 | SV2.4 3.81,39.37 6.86,39.37 | 6.35,33.02 6.35,36.83 7.62,38.1 6.86,38.86 6.86,39.37 | 6.86,39.37 6.86,44.96 v7.62,45.72
  Bottom 0.406: v12.7,25.4 21.59,25.4 21.59,25.15 v18.67,22.23 | v7.62,45.72 10.16,45.72
PD2  (via drill 0.38)  (1 unrouted)
  Top 0.203: 21.91,23.18 21.27,23.18 20.64,22.54 v20.64,21.27
  Bottom 0.203: v20.64,21.27 20.32,20.95 20.32,19.05 17.78,16.51 12.7,16.51 12.7,14.92 14.29,13.34 23.18,13.34 23.18,13.65 24.45,14.92 26.67,14.92 26.67,2.54 26.35,2.22 9.84,2.22 9.84,3.81 J2.3
PD4  (via drill 0.6)
  Top 0.406: IC1.2 19.78,25.75 20.32,26.29 20.32,38.1 21.59,39.37 25.4,39.37 26.67,40.64 26.67,44.45 27.94,45.72 27.94,55.88 v25.4,55.88 | 37.78,67.31 R8.1 37.66,66.55 v36.45,66.55
  Bottom 0.406: v25.4,55.88 25.4,64.77 26.67,66.04 35.94,66.04 v36.45,66.55
PD5  (via drill 0.6)
  Top 0.254: IC1.9 12.7,23.91 12.7,24.13 13.44,24.87 13.97,24.87
  Top 0.406: R11.1 39.18,60.77 v39.24,60.83 | v12.7,29.21 13.97,27.94 13.97,24.87
  Bottom 0.406: v39.24,60.83 39.5,60.83 40.64,59.69 40.64,55.88 39.37,54.61 26.67,54.61 25.4,53.34 25.4,48.26 22.86,45.72 22.86,40.64 24.13,39.37 24.13,38.1 22.86,36.83 13.97,36.83 11.43,34.29 12.7,33.02 v12.7,29.21
RST  (via drill 0.6)
  Top 0.254: R2(SMD).1 18.44,48.45 C4.2 | 13.06,53.34 13.06,53.87 SW2.2
  Top 0.406: 18.95,47.94 C4.2 19.05,48.26 v20.32,49.53 | R2(SMD).1 16.89,50.42 13.97,53.34 13.06,53.34 | v24.13,49.53 24.13,45.72 25.4,44.45 v25.4,43.18 | IC1.29 22.09,20.7 23.5,20.7 23.88,20.32 27.94,20.32 31.75,24.13 31.75,25.4 ICSP-PROG-HEADER.5 35.94,27.94 v37.21,29.21
  Bottom 0.406: v20.32,49.53 v24.13,49.53 | v25.4,43.18 29.21,39.37 33.53,39.37 37.21,35.69 v37.21,29.21
RX
  Top 0.406: IC1.30 22.14,21.59 24.13,21.59 24.77,22.23 24.77,28.57 24.13,29.21 FTDI-SERIAL-HEADER.5
SCK  (via drill 0.51, 0.6)
  Top 0.406: v22.86,62.23 22.54,62.23 R1.2 | SV3.3 v3.81,17.78 5.08,16.51 5.08,15.24 6.35,13.97 13.97,13.97 14.98,14.98 IC1.17 14.98,18.79 15.24,19.05 15.88,19.05 16,19.18 v16.51,19.18
  Bottom 0.406: v22.86,62.23 19.05,62.23 15.24,58.42 15.24,48.26 13.97,46.99 6.35,46.99 5.08,45.72 5.08,43.18 3.81,41.91 4.95,40.77 4.95,36.96 v5.08,36.83 5.08,19.05 v3.81,17.78 | ICSP-PROG-HEADER.3 31.75,26.67 30.48,25.4 29.21,25.4 27.94,26.67 25.02,26.67 22.86,24.51 22.1,24.51 16.89,18.92 16.76,18.92 v16.51,19.18
SEN_A
  Top 0.406: R5.1 44.83,54.99 46.99,57.15 50.8,57.15 IC4.1
SEN_B  (via drill 0.51)
  Top 0.254: v63.5,52.45 63.5,48.26 61.72,46.48 R6.1
  Bottom 0.254: v63.5,52.45 63.5,53.34 64.77,54.61 67.31,54.61 71.12,58.42 IC4.15
TX  (via drill 0.6)
  Top 0.406: FTDI-SERIAL-HEADER.4 26.67,33.02 25.4,31.75 v25.4,30.48 | 22.17,22.23 IC1.31 23.84,22.32 24.13,22.61 24.13,23.88 22.86,25.15 v22.86,30.48
  Bottom 0.406: v25.4,30.48 v22.86,30.48
VCC
  Top 0.406: 67.53,15.24 66.31,14.02 D9.C | LED5.C arc-45 71.64,11.13 67.53,15.24 | 67.53,15.24 66.14,15.24 arc-45 65.97,15.31 60.96,20.32 60.96,23.77 arc45 60.89,23.95 K2.1

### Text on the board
tPlace: greenhouse | power | project | pcb | h-bridge | power | opto | brent | dave | jarred | sck | let there be light | rst | lcd | opto | fan | dtr | FTDI | rx | tx | +5v | gnd | water pump | relay | +5v | gnd | ICSP | miso | sck | rst | High Voltage | bulb | vreg | High Voltage | 328p | photoresistor #1 | water level | temp sensor | photoresistor #2 | soil level | servo | pd2 | pc0 | pc1 | pb1 | pc3 | pc2
bPlace: <3 | oshw | Greenhouse Project / brent/dave/jarred

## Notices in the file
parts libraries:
SparkFun-Aesthetics: Licensing: Creative Commons ShareAlike 4.0 International - https://creativecommons.org/licenses/by-sa/4.0
